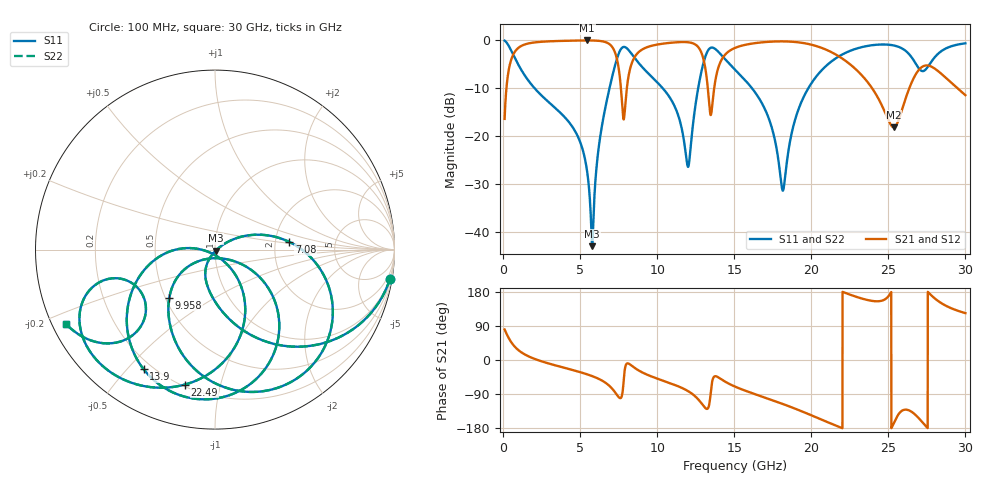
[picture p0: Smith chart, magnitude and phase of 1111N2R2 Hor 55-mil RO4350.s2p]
# GHz S MA R 50
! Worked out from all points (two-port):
!   3201 points, 100 MHz to 30 GHz, reference 50 ohm
!   highest |S21| = -0.06 dB at 5.463 GHz (marker M1); lowest = -18.2 dB at 25.35 GHz (marker M2)
!   |S21| within 3 dB of the highest: 651.2 MHz to 7.316 GHz (6.665 GHz wide, 167 % of centre); 14.4 GHz to 21.63 GHz (7.227 GHz wide, 40.1 % of centre)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
!   lowest |S11| = -43.0 dB at 5.781 GHz (marker M3), VSWR 1.01, Z = 50.5 - j0.536 ohm
!   |S11| at or under -10 dB: 2.039 GHz to 6.907 GHz (4.868 GHz wide, 109 % of centre); 10.35 GHz to 12.66 GHz (2.306 GHz wide, 20 % of centre); 16.15 GHz to 19.81 GHz (3.666 GHz wide, 20.4 % of centre)
!   |S22| runs from -43.0 to -0.1 dB; largest |S21 - S12| = 0
!   S11 on the Smith chart (normalised r, x): 100 MHz: 1, -12; 7.08 GHz: 2.39, +0.25; 9.958 GHz: 0.52, -0.33; 13.9 GHz: 0.17, -0.56; 22.49 GHz: 0.21, -0.78; 30 GHz: 0.04, -0.24
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0.1  0.9885 -9.5  0.1511 80.5  0.1511 80.5  0.9885 -9.5
1.548281  0.3976 -78.1  0.9163 11.7  0.9163 11.7  0.3976 -78.1
5.089563  0.07909 -120.3  0.9924 -33.1  0.9924 -33.1  0.07909 -120.3
5.463312  0.04183 -120.8  0.9933 -37.9  0.9933 -37.9  0.04183 -120.8
5.781  0.007105 -48.4  0.9923 -42.5  0.9923 -42.5  0.007105 -48.4
7.079781  0.416 5.9  0.85 -75.7  0.85 -75.7  0.416 5.9
8.0235  0.8255 -73.7  0.3074 -9.7  0.3074 -9.7  0.8255 -73.7
9.957656  0.3696 -133.5  0.8972 -48.4  0.8972 -48.4  0.3696 -133.5
10.06978  0.3543 -135.1  0.904 -50.0  0.904 -50.0  0.3543 -135.1
12.00394  0.04772 -88.8  0.9513 -82.1  0.9513 -82.1  0.04772 -88.8
13.03175  0.6013 -54.0  0.607 -122.5  0.607 -122.5  0.6013 -54.0
13.47091  0.8331 -91.6  0.1658 -87.9  0.1658 -87.9  0.8331 -91.6
13.90072  0.7759 -120.9  0.4739 -44.3  0.4739 -44.3  0.7759 -120.9
15.05  0.4937 -155.8  0.8308 -70.2  0.8308 -70.2  0.4937 -155.8
17.12431  0.1706 177.4  0.9589 -101.0  0.9589 -101.0  0.1706 177.4
18.15213  0.02695 -117.5  0.9713 -116.0  0.9713 -116.0  0.02695 -117.5
20.03956  0.3616 -62.3  0.8946 -146.5  0.8946 -146.5  0.3616 -62.3
22.48763  0.7706 -102.6  0.565 172.8  0.565 172.8  0.7706 -102.6
25.01978  0.8967 -141.9  0.1449 169.0  0.1449 169.0  0.8967 -141.9
25.34681  0.8812 -147.2  0.1233 -167.7  0.1233 -167.7  0.8812 -147.2
27.28097  0.4768 -147.0  0.5368 -167.5  0.5368 -167.5  0.4768 -147.0
30  0.9279 -153.5  0.267 123.7  0.267 123.7  0.9279 -153.5
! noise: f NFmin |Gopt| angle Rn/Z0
0.1  0.001712  0.9017  3.073  0.003811
3.417  0.01109  0.5298  27.99  0.003934
6.743  0.05914  0.8021  48.75  0.05157
10.06  0.07452  0.779  71.38  0.04592
13.39  0.8342  0.9719  90.43  3.368
16.7  0.08265  0.7039  109.5  0.01936
20.03  0.1106  0.736  124.2  0.01982
23.35  0.3054  0.8826  139.9  0.06822
26.67  0.7185  0.941  155.4  0.1266
30  0.4373  0.8982  167.7  0.01341
